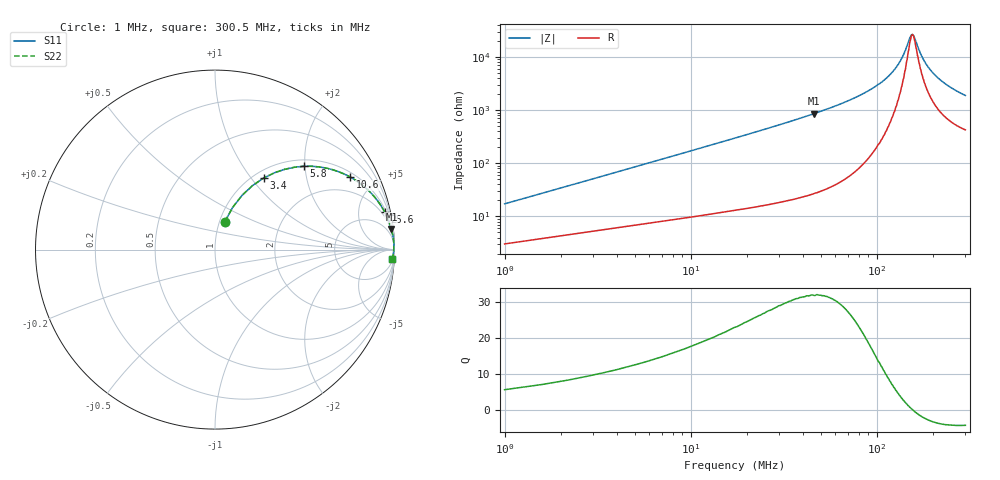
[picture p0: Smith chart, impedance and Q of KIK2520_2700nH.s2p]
!version-2
!date-01.2022
!Series
# MHz S RI R 50
!Freq ReS11 ImS11 ReS21 ImS21 ReS12 ImS12 ReS22 ImS22
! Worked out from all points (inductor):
!   500 points, 1 MHz to 300.5 MHz, reference 50 ohm
!   read as one part in series: L = 2.7 uH near 2.2 MHz
!   highest Q = 31.9 at 46 MHz (marker M1), where L = 2.96 uH
!   self-resonance near 156 MHz
!   S11 on the Smith chart (normalised r, x): 1 MHz: 1.06, +0.34; 3.4 MHz: 1.11, +1.15; 5.8 MHz: 1.15, +1.97; 10.6 MHz: 1.20, +3.61; 25.6 MHz: 1.33, +8.93; 300.5 MHz: 9, -37
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1  0.0551 0.1556  0.9449 -0.1556  0.9449 -0.1556  0.0551 0.1556
3.4  0.2708 0.3985  0.7292 -0.3985  0.7292 -0.3985  0.2708 0.3985
5.8  0.4944 0.4641  0.5056 -0.4641  0.5056 -0.4641  0.4944 0.4641
8.2  0.6524 0.4459  0.3476 -0.4459  0.3476 -0.4459  0.6524 0.4459
10.6  0.7541 0.4039  0.2459 -0.4039  0.2459 -0.4039  0.7541 0.4039
16.6  0.8799 0.3036  0.1201 -0.3036  0.1201 -0.3036  0.8799 0.3036
25.6  0.9453 0.2098  0.0547 -0.2098  0.0547 -0.2098  0.9453 0.2098
46  0.983 0.1144  0.017 -0.1144  0.017 -0.1144  0.983 0.1144
51.4  0.9866 0.1004  0.0134 -0.1004  0.0134 -0.1004  0.9866 0.1004
101  0.9965 0.0334  0.00352 -0.0334  0.00352 -0.0334  0.9965 0.0334
116  0.9969 0.0228  0.00314 -0.0228  0.00314 -0.0228  0.9969 0.0228
131  0.9969 0.0134  0.00315 -0.0134  0.00315 -0.0134  0.9969 0.0134
140  0.9967 0.00832  0.00329 -0.00832  0.00329 -0.00832  0.9967 0.00832
151  0.9964 0.00244  0.00359 -0.00244  0.00359 -0.00244  0.9964 0.00244
154  0.9963 0.000975  0.00369 -0.000975  0.00369 -0.000975  0.9963 0.000975
158  0.9962 -0.000745  0.00382 0.000745  0.00382 0.000745  0.9962 -0.000745
169  0.9957 -0.00594  0.00429 0.00594  0.00429 0.00594  0.9957 -0.00594
178  0.9953 -0.00979  0.00472 0.00979  0.00472 0.00979  0.9953 -0.00979
201  0.994 -0.0188  0.00602 0.0188  0.00602 0.0188  0.994 -0.0188
223  0.9925 -0.0268  0.00755 0.0268  0.00755 0.0268  0.9925 -0.0268
251  0.9903 -0.0358  0.00974 0.0358  0.00974 0.0358  0.9903 -0.0358
300.5  0.9857 -0.0502  0.0143 0.0502  0.0143 0.0502  0.9857 -0.0502
